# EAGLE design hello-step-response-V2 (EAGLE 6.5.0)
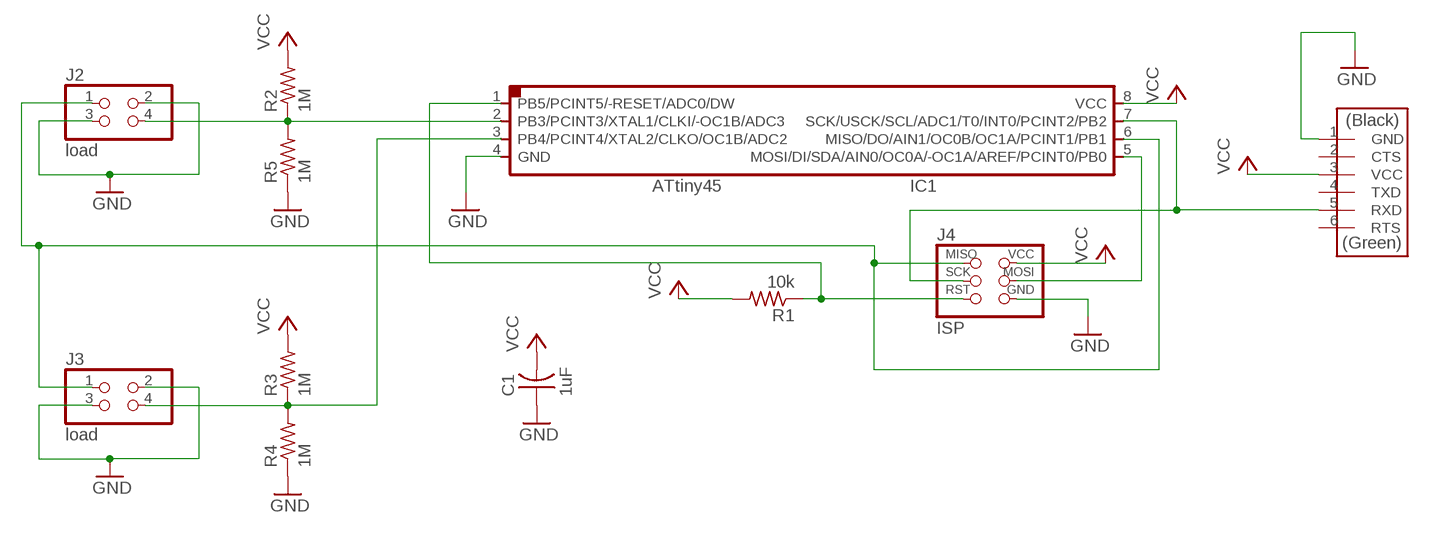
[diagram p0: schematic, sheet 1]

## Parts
C1  1uF  CAP-US1206FAB  [C1206FAB]
IC1  ATTINY45  ATTINY45SI  [SOIC8]
J1  FTDI  FTDI-SMD-HEADER  [1X06SMD]
J2  load  PINHD-2X2-SMD  [2X02SMD]
J3  load  PINHD-2X2-SMD  [2X02SMD]
J4  ISP  AVRISPSMD  [2X03SMD]
R1  10k  RES-US1206FAB  [R1206FAB]
R2  1M  RES-US1206FAB  [R1206FAB]
R3  1M  RES-US1206FAB  [R1206FAB]
R4  1M  RES-US1206FAB  [R1206FAB]
R5  1M  RES-US1206FAB  [R1206FAB]

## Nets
GND: C1.1 IC1.4(GND) J1.1(GND) J2.2 J2.3 J3.2 J3.3 J4.6(GND) R4.1 R5.1
MISO: IC1.6(MISO/DO/AIN1/OC0B/OC1A/PCINT1/PB1) J2.1 J3.1 J4.1(MISO)
MOSI: IC1.5(MOSI/DI/SDA/AIN0/OC0A/-OC1A/AREF/PCINT0/PB0) J4.4(MOSI)
N$1: IC1.3(PB4/PCINT4/XTAL2/CLKO/OC1B/ADC2) J3.4 R3.1 R4.2
N$2: IC1.2(PB3/PCINT3/XTAL1/CLKI/-OC1B/ADC3) J2.4 R2.1 R5.2
RST: IC1.1(PB5/PCINT5/-RESET/ADC0/DW) J4.5(RST) R1.1
SCK: IC1.7(SCK/USCK/SCL/ADC1/T0/INT0/PCINT2/PB2) J1.5(RXD) J4.3(SCK)
VCC: C1.2 IC1.8(VCC) J1.3(VCC) J4.2(VCC) R1.2 R2.2 R3.2
Unconnected: J1.2(CTS) J1.4(TXD) J1.6(RTS)

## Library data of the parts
C1 = fab:CAP-US
IC1 = fab:ATTINY45
J1 = fab:FTDI-SMD-HEADER
J2 J3 = fab:PINHD-2X2-SMD
J4 = fab:AVRISP
R1-R5 = fab:RES-US: Resistor (US Symbol)

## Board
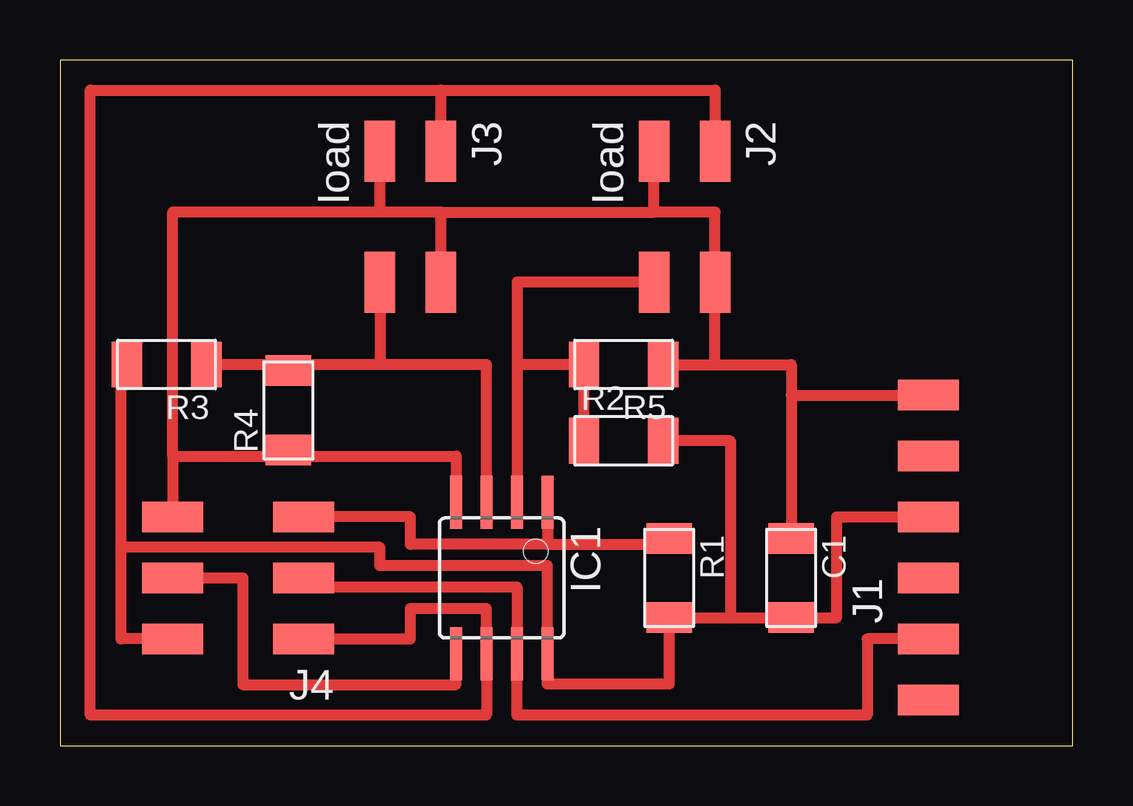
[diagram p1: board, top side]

Size 42.22 x 28.56 mm. Coordinates in mm from the lower left corner, seen from the top.
Outline: 0,0 42.22,0 42.22,28.56 0,28.56 0,0
Copper layers (1*16): Top 0.035mm / dielectric 1.5mm / Bottom 0.035mm
Design rules "design-rules-fablab": minimum track width 18mil, minimum drill 24mil, track to track 0.4mm, track to pad 0.4mm, pad to pad 0.4mm, via to via 0.4mm, smd to smd 8mil, copper to edge 1mil, drill to drill 8mil, minimum pad ring 10mil, minimum via ring 8mil, stop-mask expansion 4mil, vias tented up to drill 0mil, thermal gap 10mil

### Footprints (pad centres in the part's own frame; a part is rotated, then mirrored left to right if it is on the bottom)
C1206FAB = smd 1.27 x 1.905: 1 -1.651,0; 2 1.651,0
SOIC8 = smd 0.5 x 2.2: 1 -1.905,-3.154; 2 -0.645,-3.154; 3 0.625,-3.154; 4 1.895,-3.154; 5 1.905,3.154; 6 0.635,3.154; 7 -0.635,3.154; 8 -1.905,3.154
1X06SMD = smd 2.54 x 1.27: 1 0,6.35; 2 0,3.81; 3 0,1.27; 4 0,-1.27; 5 0,-3.81; 6 0,-6.35
2X02SMD = smd 2.54 x 1.27: 1 -2.54,1.27; 2 2.92,1.27; 3 -2.54,-1.27; 4 2.92,-1.27
2X03SMD = smd 2.54 x 1.27: 1 -2.54,2.54; 2 2.92,2.54; 3 -2.54,0; 4 2.92,0; 5 -2.54,-2.54; 6 2.92,-2.54
R1206FAB = smd 1.27 x 1.905: 1 -1.651,0; 2 1.651,0

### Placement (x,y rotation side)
C1  30.48,6.99 270 top
IC1  18.41,6.99 180 top
J1  36.2,8.26 0 top
J2  26.04,22.22 270 top
J3  14.61,22.22 270 top
J4  7.62,6.99 180 top
R1  25.4,6.99 270 top
R2  23.49,12.7 0 top
R3  4.45,15.88 180 top
R4  9.53,13.97 90 top
R5  23.49,15.88 180 top

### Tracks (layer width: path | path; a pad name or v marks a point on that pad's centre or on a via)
GND
  Top 0.457: 30.48,14.61 C1.1 | 4.7,12.06 9.53,12.06 | 9.53,12.06 16.52,12.06 IC1.4 | 4.7,12.06 J4.6 | 15.88,22.22 13.34,22.22 | 13.34,22.22 J3.3 | 24.76,22.22 27.3,22.22 J2.2 27.3,15.88 | 24.76,22.22 J2.3 | 15.88,22.22 24.76,22.22 | 36.2,14.99 J1.1 30.48,14.61 | 4.7,12.06 4.7,22.22 13.34,22.22 | J3.2 15.88,22.22 | R4.1 9.53,12.06 | R5.1 27.3,15.88 | 27.3,15.88 30.48,15.88 30.48,14.61
MISO
  Top 0.457: 9.53,4.45 J4.1 14.61,4.45 14.61,5.71 17.78,5.71 IC1.6 17.78,1.27 1.27,1.27 1.27,27.3 15.88,27.3 | J3.1 15.88,27.3 | 15.88,27.3 27.3,27.3 J2.1
MOSI
  Top 0.457: J4.4 7.62,6.99 7.62,2.54 16.51,2.54 IC1.5
N$1
  Top 0.457: IC1.3 17.78,10.14 17.78,15.88 13.34,15.88 | 13.34,15.88 9.53,15.88 | 9.53,15.88 R3.1 | J3.4 13.34,15.88 | R4.2 9.53,15.88
N$2
  Top 0.457: J2.4 19.06,19.3 19.06,15.88 | 19.06,15.88 IC1.2 | R2.1 R5.2 19.06,15.88
RST
  Top 0.457: 24.76,8.64 R1.1 25.4,8.38 20.32,8.38 | 24.76,8.64 24.76,8.26 | 24.76,8.89 24.76,8.64 | IC1.1 20.32,8.38 | 20.32,8.38 14.61,8.38 14.61,9.53 J4.5
SCK
  Top 0.457: J1.5 33.66,4.45 33.66,1.27 19.05,1.27 IC1.7 19.05,6.6 10.16,6.6 J4.3
VCC
  Top 0.457: J4.2 2.54,4.45 2.54,8.26 | 27.94,5.33 R1.2 25.4,2.56 20.32,2.56 IC1.8 20.32,7.49 13.34,7.49 13.34,8.26 2.54,8.26 | 27.94,5.33 C1.2 32.39,5.33 32.39,9.53 J1.3 | R3.2 2.54,15.88 2.54,8.26 | 27.94,5.33 27.94,12.7 R2.2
